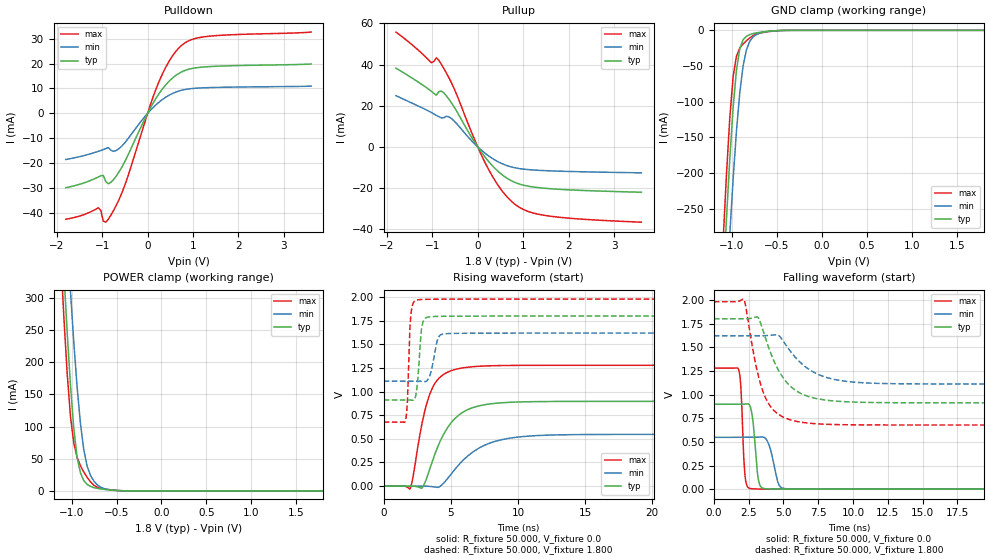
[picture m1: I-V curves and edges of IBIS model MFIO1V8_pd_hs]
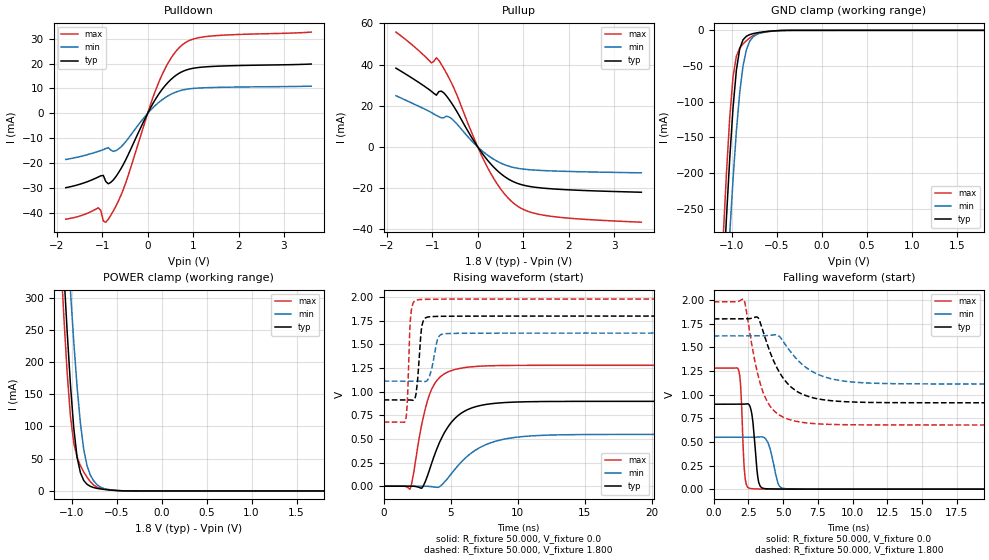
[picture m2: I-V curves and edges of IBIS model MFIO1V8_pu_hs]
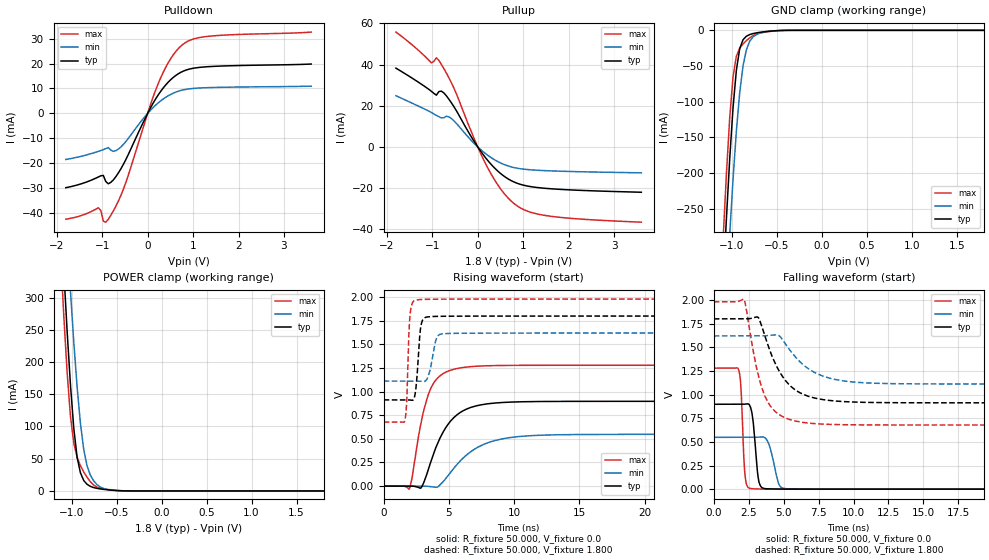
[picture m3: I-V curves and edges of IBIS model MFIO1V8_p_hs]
| IBIS file lpc55s6x_vfbga98.ibs
[IBIS Ver]   5.0
[File name]   lpc55s6x_vfbga98.ibs
[File Rev]   1.0
[Date]   May 25,2020
[Notes]   Rev History
|   1.0  initial release
[Disclaimer]   The model given below represents a 98-pin package.
[Copyright]   Copyright NXP 2020
|   Component lpc55s6x:vfbga98
[Component] lpc55s6x
[Manufacturer] NXP
[Package]
|   typ   min   max
R_pkg   0.1209   0.044925   0.28644
L_pkg   2.048e-9   9.518e-10   5.863e-9
C_pkg   3.001e-13   1.858e-13   5.678e-13
[Pin]   Signal_name   model_name   R_pin   L_pin   C_pin
G2   VDDA   POWER   NA   NA   NA
N7   USB1_3V3   POWER   NA   NA   NA
A3   USB0_3V3   POWER   NA   NA   NA
A5   VDD   POWER   NA   NA   NA
A9   VDD   POWER   NA   NA   NA
A13   VDD   POWER   NA   NA   NA
M1   VDD   POWER   NA   NA   NA
M9   VDD_PMU   POWER   NA   NA   NA
N6   USB1_DM   NC   0.094006   1.426e-9   2.165e-13
M6   USB1_DP   NC   0.094615   1.516e-9   2.317e-13
N9   FB   NC   0.12218   1.681e-9   2.209e-13
N11   LX   NC   0.06538   1.432e-9   3.1e-13
L12   P0_0   gpio1v8   0.094413   1.591e-9   2.392e-13
F5   P0_1   gpio1v8   0.09009   1.63e-9   3.407e-13
B11   P0_2   gpio1v8   0.10271   1.839e-9   2.924e-13
F8   P0_3   gpio1v8   0.1454   2.708e-9   3.901e-13
E7   P0_4   gpio1v8   0.091626   1.515e-9   3.275e-13
A7   P0_5   gpio1v8   0.12923   2.076e-9   2.188e-13
B7   P0_6   gpio1v8   0.11077   1.654e-9   2.153e-13
G5   P0_7   gpio1v8   0.13963   2.496e-9   4.691e-13
M2   P0_8   gpio1v8   0.095249   1.692e-9   2.933e-13
L13   P0_9   gpio1v8   0.15164   2.569e-9   2.247e-13
F2   P0_10   gpio1v8   0.12482   2.207e-9   3.527e-13
F1   P0_11   gpio1v8   0.13661   2.235e-9   2.226e-13
E2   P0_12   gpio1v8   0.10697   1.857e-9   3.137e-13
C12   P0_13   iicgpio1v8   0.15036   2.528e-9   2.486e-13
C13   P0_14   iicgpio1v8   0.15468   2.443e-9   2.364e-13
L2   P0_15   gpio1v8   0.098205   1.674e-9   2.761e-13
J2   P0_16   gpio1v8   0.12449   2.514e-9   2.708e-13
G3   P0_17   gpio1v8   0.075726   1.285e-9   2.687e-13
H9   P0_18   gpio1v8   0.087847   1.562e-9   3.542e-13
E6   P0_19   gpio1v8   0.083442   1.458e-9   2.858e-13
B12   P0_20   gpio1v8   0.14629   2.14e-9   2.464e-13
A12   P0_21   gpio1v8   0.12809   1.906e-9   1.918e-13
E9   P0_22   gpio1v8   0.094505   1.588e-9   3.718e-13
J1   P0_23   gpio1v8   0.13195   1.94e-9   2.141e-13
E12   P0_24   gpio1v8   0.091918   1.666e-9   2.453e-13
A11   P0_25   gpio1v8   0.11529   1.718e-9   1.949e-13
H12   P0_26   gpio1v8   0.081253   1.5e-9   2.767e-13
N2   P0_27   gpio1v8   0.13095   2.225e-9   3.428e-13
F13   P0_28   gpio1v8   0.13767   2.192e-9   2.158e-13
H8   P0_29   gpio1v8   0.15886   3.15e-9   5.678e-13
E5   P0_30   gpio1v8   0.086667   1.519e-9   3.383e-13
L1   P0_31   gpio1v8   0.15272   2.424e-9   2.59e-13
E1   P1_0   gpio1v8   0.14644   2.463e-9   2.597e-13
G11   P1_1   gpio1v8   0.096065   1.69e-9   3.188e-13
G12   P1_2   gpio1v8   0.12798   2.099e-9   2.352e-13
G13   P1_3   gpio1v8   0.12828   1.937e-9   2.153e-13
B2   P1_4   gpio1v8   0.096863   1.598e-9   2.988e-13
M5   P1_5   gpio1v8   0.094289   1.603e-9   3.053e-13
H5   P1_6   gpio1v8   0.16673   3.191e-9   4.881e-13
J5   P1_7   gpio1v8   0.12619   2.354e-9   3.979e-13
A6   P1_8   gpio1v8   0.28644   5.863e-9   4.62e-13
C1   P1_9   gpio1v8   0.1694   3.073e-9   3.031e-13
J7   P1_10   gpio1v8   0.08793   1.355e-9   3.087e-13
G6   P1_11   gpio1v8   0.15151   2.536e-9   5.272e-13
F12   P1_12   gpio1v8   0.082887   1.462e-9   2.268e-13
B3   P1_13   gpio1v8   0.11404   1.893e-9   2.97e-13
L7   P1_14   gpio1v8   0.18217   3.548e-9   3.635e-13
B6   P1_15   gpio1v8   0.12901   2.443e-9   3.381e-13
C7   P1_16   gpio1v8   0.072915   1.186e-9   2.322e-13
J9   P1_17   gpio1v8   0.10787   1.748e-9   3.803e-13
G9   P1_18   gpio1v8   0.091968   1.458e-9   3.094e-13
H13   P1_19   gpio1v8   0.12429   2.047e-9   2.027e-13
C2   P1_20   gpio1v8   0.096736   1.471e-9   2.029e-13
M7   P1_21   gpio1v8   0.14632   2.946e-9   3.43e-13
M8   P1_22   gpio1v8   0.076897   1.014e-9   2.527e-13
J8   P1_23   gpio1v8   0.085096   1.345e-9   3.077e-13
F6   P1_24   gpio1v8   0.13441   2.357e-9   4.172e-13
B8   P1_25   gpio1v8   0.10461   2.067e-9   3.287e-13
E13   P1_26   gpio1v8   0.12992   1.953e-9   2.102e-13
E8   P1_27   gpio1v8   0.11191   1.807e-9   3.572e-13
A8   P1_28   gpio1v8   0.21716   4.383e-9   3.836e-13
G8   P1_29   gpio1v8   0.15479   2.956e-9   4.522e-13
F9   P1_30   gpio1v8   0.093936   1.556e-9   3.54e-13
H6   P1_31   gpio1v8   0.14695   2.973e-9   5.442e-13
J6   RESETN   gpio1v8   0.08999   1.312e-9   3.328e-13
A1   USB0_DM   NC   0.17463   2.687e-9   2.917e-13
A2   USB0_DP   NC   0.16587   2.364e-9   2.831e-13
N13   VBAT_DCDC   NC   0.044925   1.39e-9   3.067e-13
M13   VBAT_PMU   NC   0.11627   1.679e-9   2.076e-13
N8   VBUS   NC   0.076519   9.518e-10   1.858e-13
H1   VREFN   NC   0.12485   1.889e-9   2.171e-13
G1   VREFP   NC   0.12475   1.856e-9   2.204e-13
J12   XTAL32K_N   NC   0.11411   1.691e-9   2.046e-13
J13   XTAL32K_P   NC   0.13248   1.96e-9   2.273e-13
M3   XTAL32M_N   NC   0.15178   2.164e-9   3.058e-13
N3   XTAL32M_P   NC   0.14758   1.994e-9   3.19e-13
B5   VSS   GND   NA   NA   NA
B9   VSS   GND   NA   NA   NA
B13   VSS   GND   NA   NA   NA
N1   VSS   GND   NA   NA   NA
H2   VSSA   GND   NA   NA   NA
N5   USB1_VSS   GND   NA   NA   NA
N12   VSS_DCDC   GND   NA   NA   NA
M12   VSS_DCDC   GND   NA   NA   NA
M11   VSS_PMU   GND   NA   NA   NA
B1   USB0_VSS   GND   NA   NA   NA
|   Model Selector
[Model Selector] gpio1v8
MFIO1V8_pd_hs  EPUN=1 EPD=1 EHS=1
MFIO1V8_pd_ls  EPUN=1 EPD=1 EHS=0
MFIO1V8_pu_hs  EPUN=0 EPD=0 EHS=1
MFIO1V8_pu_ls  EPUN=0 EPD=0 EHS=0
MFIO1V8_p_hs  EPUN=1 EPD=0 EHS=1
MFIO1V8_p_ls  EPUN=1 EPD=0 EHS=0
MFIO1V8_r_hs  EPUN=0 EPD=1 EHS=1
MFIO1V8_r_ls  EPUN=0 EPD=1 EHS=0
[Model Selector] iicgpio1v8
IIC1V8_pd_hs  EGP=1 EPUN=1 EPD=1 EHS=1
IIC1V8_pd_ls  EGP=1 EPUN=1 EPD=1 EHS=0
IIC1V8_p_hs  EGP=1 EPUN=1 EPD=0 EHS=1
IIC1V8_p_ls  EGP=1 EPUN=1 EPD=0 EHS=0
IIC1V8_pu_hs  EGP=1 EPUN=0 EPD=0 EHS=1
IIC1V8_pu_ls  EGP=1 EPUN=0 EPD=0 EHS=0
IIC1V8_r_hs  EGP=1 EPUN=0 EPD=1 EHS=1
IIC1V8_r_ls  EGP=1 EPUN=0 EPD=1 EHS=0
IIC1V8_pd_iic_hs  EGP=0 ECS=0 EPUN=1 EPD=1
IIC1V8_p_iic_hs  EGP=0 ECS=0 EPUN=1 EPD=0
IIC1V8_pu_iic_hs  EGP=0 ECS=0 EPUN=0 EPD=0
IIC1V8_r_iic_hs  EGP=0 ECS=0 EPUN=0 EPD=1
IIC1V8_pd_iic_pu_hs  EGP=0 ECS=1 EPUN=1 EPD=1  SSEL=1
IIC1V8_p_iic_pu_hs  EGP=0 ECS=1 EPUN=1 EPD=0  SSEL=1
IIC1V8_pu_iic_pu_hs  EGP=0 ECS=1 EPUN=0 EPD=0  SSEL=1
IIC1V8_r_iic_pu_hs  EGP=0 ECS=1 EPUN=0 EPD=1  SSEL=1
| Models and submodels in the file (24): MFIO1V8_pd_hs (I/O), MFIO1V8_pd_ls (I/O), MFIO1V8_pu_hs (I/O), MFIO1V8_pu_ls (I/O), MFIO1V8_p_hs (I/O), MFIO1V8_p_ls (I/O), MFIO1V8_r_hs (I/O), MFIO1V8_r_ls (I/O), IIC1V8_pd_hs (I/O), IIC1V8_pd_ls (I/O), IIC1V8_p_hs (I/O), IIC1V8_p_ls (I/O), IIC1V8_pu_hs (I/O), IIC1V8_pu_ls (I/O), IIC1V8_r_hs (I/O), IIC1V8_r_ls (I/O), IIC1V8_pd_iic_hs (I/O_open_drain), IIC1V8_p_iic_hs (I/O_open_drain), IIC1V8_pu_iic_hs (I/O_open_drain), IIC1V8_r_iic_hs (I/O_open_drain), IIC1V8_pd_iic_pu_hs (I/O_open_drain), IIC1V8_p_iic_pu_hs (I/O_open_drain), IIC1V8_pu_iic_pu_hs (I/O_open_drain), IIC1V8_r_iic_pu_hs (I/O_open_drain)
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|   Model MFIO1V8_pd_hs
[Model] MFIO1V8_pd_hs
Model_type I/O
Polarity   Non-Inverting
Enable   Active-Low
Vinl =  0.540V
Vinh =  1.260V
Vmeas =  0.900V
Cref =  0.0F
Rref =  100.000
Vref =  0.0V
C_comp   2.019pF   1.989pF   2.068pF
C_comp_pullup   1.198pF   1.161pF   1.251pF
C_comp_pulldown   0.670pF   0.661pF   0.684pF
[Model Spec]
Vinh   1.260V   1.134V   1.386V
Vinl   0.540V   0.486V   0.594V
Vmeas   0.900V   0.810V   0.990V
Vref   0.0V   0.0V   0.0V
Cref   0.0F   0.0F   0.0F
Rref   100.000   100.000   100.000
[Temperature Range]   25.000   0.125k   -40.000
[Voltage Range]   1.800V   1.620V   1.980V
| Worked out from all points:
|   slope of the pulldown table from 0 to 0.27 V, typ, clamps not added: 32.2 ohm
|   slope of the pullup table from 0 to 0.27 V, typ, clamps not added: 34.3 ohm
|   GND clamp passes 1 mA (typ) near -0.56 V on its own axis
|   POWER clamp passes 1 mA (typ) near -0.54 V on its own axis
|   rising waveform, R_fixture 50.000, V_fixture 0.0: 20-80 % time 1.89ns typ, 2.69ns min, 1.21ns max; typ from 0 V to 0.897 V
|   rising waveform, R_fixture 50.000, V_fixture 1.800: 20-80 % time 276ps typ, 422ps min, 194ps max; typ from 0.912 V to 1.8 V
|   falling waveform, R_fixture 50.000, V_fixture 0.0: 20-80 % time 315ps typ, 502ps min, 217ps max; typ from 0.897 V to 0 V
|   falling waveform, R_fixture 50.000, V_fixture 1.800: 20-80 % time 1.84ns typ, 2.3ns min, 1.28ns max; typ from 1.8 V to 0.912 V
[Pulldown]
|Voltage   I(typ)   I(min)   I(max)
-1.8V     -29.75mA   -18.45mA   -42.39mA
-1.085V   -25.48mA   -15.2mA    -37.79mA
-1.03V    -24.99mA   -14.87mA   -38.88mA
-975mV    -24.83mA   -14.51mA   -43.15mA
-865mV    -28.18mA   -13.68mA   -42.43mA
-700mV    -25.38mA   -14.92mA   -37.23mA
-480mV    -18.54mA   -11.29mA   -27.73mA
235mV     7.474mA    4.265mA    12.03mA
510mV     13.55mA    7.648mA    22.01mA
785mV     16.96mA    9.446mA    27.8mA
1.39V     18.81mA    10.38mA    31.01mA
3.6V      19.8mA     10.93mA    32.61mA
[Pullup]
|Voltage   I(typ)   I(min)   I(max)
-1.8V     38.29mA    24.9mA     55.82mA
-1.02V    27.05mA    16.71mA    40.87mA
-910mV    25.14mA    15.31mA    43.32mA
-855mV    26.89mA    14.69mA    42.04mA
-745mV    26.24mA    14.22mA    38.06mA
-580mV    21.45mA    13.82mA    31.22mA
190mV     -5.761mA   -3.564mA   -8.914mA
520mV     -13.24mA   -7.997mA   -20.92mA
795mV     -17.02mA   -10.03mA   -27.47mA
1.07V     -18.92mA   -10.95mA   -31.04mA
1.51V     -20.18mA   -11.56mA   -33.41mA
3.6V      -22.04mA   -12.6mA    -36.6mA
[GND_clamp]
|Voltage   I(typ)   I(min)   I(max)
-1.8V     -2.463A    -2.494A    -2.446A
-1.097V   -357.7mA   -460.7mA   -294.8mA
-1.06V    -264.9mA   -370.9mA   -202.5mA
-1.023V   -180.4mA   -286.3mA   -122.9mA
-986mV    -108.7mA   -208.9mA   -65.05mA
-949mV    -56.06mA   -141.4mA   -36.24mA
-912mV    -25.87mA   -87.65mA   -25.01mA
-875mV    -13.21mA   -49.99mA   -19.06mA
-838mV    -8.315mA   -27.44mA   -14.52mA
-764mV    -4.558mA   -9.219mA   -7.395mA
-542mV    -813.9uA   -810.7uA   -1.086mA
1.8V      0A         0A         0A
[POWER_clamp]
|Voltage   I(typ)   I(min)   I(max)
-1.8V     2.577A     2.626A     2.553A
-1.123V   442.8mA    582.7mA    371.8mA
-1.086V   342mA      487.8mA    272.2mA
-1.049V   248.2mA    396.7mA    184.1mA
-1.012V   164.7mA    310.5mA    115.9mA
-975mV    97.4mA     231.2mA    74.47mA
-938mV    52.21mA    161.5mA    52.2mA
-864mV    16.15mA    64.06mA    29.43mA
-790mV    7.073mA    24.26mA    14.23mA
-679mV    3.152mA    6.087mA    4.407mA
-494mV    590.1uA    655.5uA    758.5uA
1.8V      0A         0A         0A
[Ramp]
| variable   typ   min   max
dV/dt_r   0.538/1.890n   0.328/2.680n   0.767/1.209n
dV/dt_f   0.532/1.835n   0.305/2.291n   0.781/1.275n
R_load = 50.000
[Rising Waveform]
R_fixture= 50.000
V_fixture= 0.0
V_fixture_min= 0.0
V_fixture_max= 0.0
|time   V(typ)   V(min)   V(max)
0s        6.721nV    117.6nV    4.416nV
1.96ns    159.2uV    -62.09nV   -31.69mV
2.85ns    -21.07mV   134.7uV    661mV
3.65ns    271.3mV    -6.708mV   1.047V
4.15ns    457.1mV    -8.65mV    1.146V
4.97ns    661.3mV    117.8mV    1.218V
6.65ns    830.9mV    361.7mV    1.264V
9.15ns    884.8mV    501.2mV    1.276V
13.74ns   896.1mV    543.8mV    1.278V
100ns     896.7mV    547.4mV    1.278V
[Rising Waveform]
R_fixture= 50.000
V_fixture= 1.800
V_fixture_min= 1.620
V_fixture_max= 1.980
|time   V(typ)   V(min)   V(max)
0s        911.9mV    1.111V     677.7mV
1.63ns    911.9mV    1.111V     697.7mV
1.77ns    912.1mV    1.111V     900.3mV
2.05ns    909.6mV    1.111V     1.849V
2.42ns    983.6mV    1.111V     1.967V
2.68ns    1.419V     1.11V      1.973V
3.06ns    1.772V     1.105V     1.976V
4.08ns    1.796V     1.575V     1.978V
4.84ns    1.798V     1.614V     1.979V
100ns     1.799V     1.619V     1.979V
[Falling Waveform]
R_fixture= 50.000
V_fixture= 0.0
V_fixture_min= 0.0
V_fixture_max= 0.0
|time   V(typ)   V(min)   V(max)
0s        896.7mV    547.4mV    1.278V
1.79ns    896.7mV    547.4mV    1.258V
1.93ns    896.6mV    547.4mV    1.106V
2.24ns    898.4mV    547.4mV    142.2mV
2.74ns    796.7mV    547.3mV    4.509mV
3.2ns     100.7mV    550.1mV    1.658mV
3.81ns    3.552mV    517mV      778.9uV
4.65ns    1.171mV    54.78mV    345.8uV
5.34ns    645.9uV    3.088mV    186.5uV
100ns     14.3nV     131.2nV    8.877nV
[Falling Waveform]
R_fixture= 50.000
V_fixture= 1.800
V_fixture_min= 1.620
V_fixture_max= 1.980
|time   V(typ)   V(min)   V(max)
0s        1.799V     1.619V     1.979V
2.17ns    1.799V     1.619V     2.003V
3.18ns    1.813V     1.619V     1.21V
3.88ns    1.522V     1.623V     915.7mV
4.62ns    1.262V     1.626V     793.3mV
5.16ns    1.14V      1.527V     750mV
6.98ns    971mV      1.252V     694.9mV
9.25ns    925.2mV    1.144V     680.9mV
13.25ns   913mV      1.113V     677.9mV
100ns     911.9mV    1.111V     677.7mV
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|   Model MFIO1V8_pu_hs
[Model] MFIO1V8_pu_hs
Model_type I/O
Polarity   Non-Inverting
Enable   Active-Low
Vinl =  0.540V
Vinh =  1.260V
Vmeas =  0.900V
Cref =  0.0F
Rref =  100.000
Vref =  0.0V
C_comp   2.019pF   1.989pF   2.068pF
C_comp_pullup   1.197pF   1.159pF   1.249pF
C_comp_pulldown   0.671pF   0.662pF   0.686pF
[Model Spec]
Vinh   1.260V   1.134V   1.386V
Vinl   0.540V   0.486V   0.594V
Vmeas   0.900V   0.810V   0.990V
Vref   0.0V   0.0V   0.0V
Cref   0.0F   0.0F   0.0F
Rref   100.000   100.000   100.000
[Temperature Range]   25.000   0.125k   -40.000
[Voltage Range]   1.800V   1.620V   1.980V
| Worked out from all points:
|   slope of the pulldown table from 0 to 0.27 V, typ, clamps not added: 32.2 ohm
|   slope of the pullup table from 0 to 0.27 V, typ, clamps not added: 34.3 ohm
|   GND clamp passes 1 mA (typ) near -0.56 V on its own axis
|   POWER clamp passes 1 mA (typ) near -0.54 V on its own axis
|   rising waveform, R_fixture 50.000, V_fixture 0.0: 20-80 % time 1.89ns typ, 2.68ns min, 1.21ns max; typ from 0.001 V to 0.898 V
|   rising waveform, R_fixture 50.000, V_fixture 1.800: 20-80 % time 275ps typ, 425ps min, 197ps max; typ from 0.913 V to 1.8 V
|   falling waveform, R_fixture 50.000, V_fixture 0.0: 20-80 % time 314ps typ, 505ps min, 216ps max; typ from 0.898 V to 0.001 V
|   falling waveform, R_fixture 50.000, V_fixture 1.800: 20-80 % time 1.84ns typ, 2.3ns min, 1.27ns max; typ from 1.8 V to 0.913 V
[Pulldown]
|Voltage   I(typ)   I(min)   I(max)
-1.8V     -29.75mA   -18.45mA   -42.39mA
-1.085V   -25.48mA   -15.2mA    -37.79mA
-1.03V    -24.99mA   -14.87mA   -38.88mA
-975mV    -24.83mA   -14.51mA   -43.15mA
-865mV    -28.18mA   -13.68mA   -42.43mA
-700mV    -25.38mA   -14.92mA   -37.23mA
-480mV    -18.54mA   -11.29mA   -27.73mA
235mV     7.474mA    4.265mA    12.03mA
510mV     13.55mA    7.648mA    22.01mA
785mV     16.96mA    9.446mA    27.8mA
1.39V     18.81mA    10.38mA    31.01mA
3.6V      19.8mA     10.93mA    32.61mA
[Pullup]
|Voltage   I(typ)   I(min)   I(max)
-1.8V     38.29mA    24.9mA     55.82mA
-1.02V    27.05mA    16.71mA    40.87mA
-910mV    25.14mA    15.31mA    43.32mA
-855mV    26.89mA    14.69mA    42.04mA
-745mV    26.24mA    14.22mA    38.06mA
-580mV    21.45mA    13.82mA    31.22mA
190mV     -5.761mA   -3.564mA   -8.914mA
520mV     -13.24mA   -7.997mA   -20.92mA
795mV     -17.02mA   -10.03mA   -27.47mA
1.07V     -18.92mA   -10.95mA   -31.04mA
1.51V     -20.18mA   -11.56mA   -33.41mA
3.6V      -22.04mA   -12.6mA    -36.6mA
[GND_clamp]
|Voltage   I(typ)   I(min)   I(max)
-1.8V     -2.463A    -2.494A    -2.446A
-1.097V   -357.7mA   -460.7mA   -294.9mA
-1.06V    -264.9mA   -371mA     -202.6mA
-1.023V   -180.4mA   -286.4mA   -122.9mA
-986mV    -108.7mA   -208.9mA   -65.09mA
-949mV    -56.09mA   -141.5mA   -36.28mA
-912mV    -25.91mA   -87.68mA   -25.06mA
-875mV    -13.24mA   -50.02mA   -19.11mA
-838mV    -8.35mA    -27.47mA   -14.57mA
-764mV    -4.593mA   -9.247mA   -7.441mA
-542mV    -849.5uA   -838.5uA   -1.132mA
1.8V      0A         0A         0A
[POWER_clamp]
|Voltage   I(typ)   I(min)   I(max)
-1.8V     2.577A     2.626A     2.553A
-1.123V   442.8mA    582.7mA    371.7mA
-1.086V   342mA      487.8mA    272.2mA
-1.049V   248.2mA    396.7mA    184.1mA
-1.012V   164.7mA    310.5mA    115.9mA
-975mV    97.36mA    231.1mA    74.42mA
-938mV    52.18mA    161.5mA    52.15mA
-864mV    16.11mA    64.03mA    29.39mA
-790mV    7.037mA    24.23mA    14.18mA
-679mV    3.116mA    6.059mA    4.361mA
-494mV    554.4uA    627.7uA    712.3uA
1.8V      0A         0A         0A
[Ramp]
| variable   typ   min   max
dV/dt_r   0.538/1.890n   0.329/2.680n   0.767/1.209n
dV/dt_f   0.532/1.835n   0.305/2.290n   0.781/1.276n
R_load = 50.000
[Rising Waveform]
R_fixture= 50.000
V_fixture= 0.0
V_fixture_min= 0.0
V_fixture_max= 0.0
|time   V(typ)   V(min)   V(max)
0s        630.6uV    679.1uV    587.5uV
1.96ns    789.2uV    678.8uV    -30.05mV
2.85ns    -19.7mV    812.3uV    661.1mV
3.62ns    261mV      -5.421mV   1.04V
4.13ns    453.5mV    -9.012mV   1.145V
4.91ns    652mV      107.5mV    1.216V
6.6ns     829.9mV    358mV      1.264V
9.06ns    885.4mV    500.2mV    1.277V
13.76ns   897.4mV    545.1mV    1.28V
100ns     898mV      548.7mV    1.28V
[Rising Waveform]
R_fixture= 50.000
V_fixture= 1.800
V_fixture_min= 1.620
V_fixture_max= 1.980
|time   V(typ)   V(min)   V(max)
0s        913.3mV    1.112V     678.9mV
1.63ns    913.3mV    1.112V     698.4mV
1.75ns    913.5mV    1.112V     853.9mV
2.02ns    911.7mV    1.112V     1.814V
2.4ns     967.4mV    1.112V     1.968V
2.67ns    1.397V     1.111V     1.974V
3.06ns    1.773V     1.107V     1.977V
4.07ns    1.797V     1.574V     1.979V
4.83ns    1.798V     1.615V     1.98V
100ns     1.8V       1.62V      1.98V
[Falling Waveform]
R_fixture= 50.000
V_fixture= 0.0
V_fixture_min= 0.0
V_fixture_max= 0.0
|time   V(typ)   V(min)   V(max)
0s        898mV      548.7mV    1.28V
1.79ns    898mV      548.7mV    1.259V
1.93ns    897.9mV    548.6mV    1.108V
2.24ns    899.8mV    548.7mV    143.9mV
2.76ns    775.9mV    548.5mV    5.275mV
3.23ns    78.56mV    551.7mV    2.369mV
3.84ns    4.35mV     511.3mV    1.439mV
4.67ns    1.941mV    48.66mV    967uV
5.32ns    1.374mV    4.206mV    798.7uV
100ns     630.7uV    679.1uV    587.5uV
[Falling Waveform]
R_fixture= 50.000
V_fixture= 1.800
V_fixture_min= 1.620
V_fixture_max= 1.980
|time   V(typ)   V(min)   V(max)
0s        1.8V       1.62V      1.98V
2.16ns    1.8V       1.62V      2.006V
3.18ns    1.814V     1.62V      1.212V
3.84ns    1.538V     1.623V     928.3mV
4.62ns    1.264V     1.627V     794.8mV
5.16ns    1.142V     1.528V     751.1mV
7.03ns    970.5mV    1.249V     695.5mV
9.17ns    927.3mV    1.147V     682.3mV
13.26ns   914.4mV    1.115V     679mV
100ns     913.3mV    1.112V     678.9mV
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|   Model MFIO1V8_p_hs
[Model] MFIO1V8_p_hs
Model_type I/O
Polarity   Non-Inverting
Enable   Active-Low
Vinl =  0.540V
Vinh =  1.260V
Vmeas =  0.900V
Cref =  0.0F
Rref =  100.000
Vref =  0.0V
C_comp   2.019pF   1.989pF   2.068pF
C_comp_pullup   1.197pF   1.160pF   1.250pF
C_comp_pulldown   0.671pF   0.662pF   0.686pF
[Model Spec]
Vinh   1.260V   1.134V   1.386V
Vinl   0.540V   0.486V   0.594V
Vmeas   0.900V   0.810V   0.990V
Vref   0.0V   0.0V   0.0V
Cref   0.0F   0.0F   0.0F
Rref   100.000   100.000   100.000
[Temperature Range]   25.000   0.125k   -40.000
[Voltage Range]   1.800V   1.620V   1.980V
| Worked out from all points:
|   slope of the pulldown table from 0 to 0.27 V, typ, clamps not added: 32.2 ohm
|   slope of the pullup table from 0 to 0.27 V, typ, clamps not added: 34.3 ohm
|   GND clamp passes 1 mA (typ) near -0.56 V on its own axis
|   POWER clamp passes 1 mA (typ) near -0.54 V on its own axis
|   rising waveform, R_fixture 50.000, V_fixture 0.0: 20-80 % time 1.89ns typ, 2.68ns min, 1.21ns max; typ from 0 V to 0.897 V
|   rising waveform, R_fixture 50.000, V_fixture 1.800: 20-80 % time 278ps typ, 422ps min, 192ps max; typ from 0.913 V to 1.8 V
|   falling waveform, R_fixture 50.000, V_fixture 0.0: 20-80 % time 314ps typ, 511ps min, 215ps max; typ from 0.897 V to 0 V
|   falling waveform, R_fixture 50.000, V_fixture 1.800: 20-80 % time 1.84ns typ, 2.3ns min, 1.28ns max; typ from 1.8 V to 0.913 V
[Pulldown]
|Voltage   I(typ)   I(min)   I(max)
-1.8V     -29.75mA   -18.45mA   -42.39mA
-1.085V   -25.48mA   -15.2mA    -37.79mA
-1.03V    -24.99mA   -14.87mA   -38.88mA
-975mV    -24.83mA   -14.51mA   -43.15mA
-865mV    -28.18mA   -13.68mA   -42.43mA
-700mV    -25.38mA   -14.92mA   -37.23mA
-480mV    -18.54mA   -11.29mA   -27.73mA
235mV     7.474mA    4.265mA    12.03mA
510mV     13.55mA    7.648mA    22.01mA
785mV     16.96mA    9.446mA    27.8mA
1.39V     18.81mA    10.38mA    31.01mA
3.6V      19.8mA     10.93mA    32.61mA
[Pullup]
|Voltage   I(typ)   I(min)   I(max)
-1.8V     38.29mA    24.9mA     55.82mA
-1.02V    27.05mA    16.71mA    40.87mA
-910mV    25.14mA    15.31mA    43.32mA
-855mV    26.89mA    14.69mA    42.04mA
-745mV    26.24mA    14.22mA    38.06mA
-580mV    21.45mA    13.82mA    31.22mA
190mV     -5.761mA   -3.564mA   -8.914mA
520mV     -13.24mA   -7.997mA   -20.92mA
795mV     -17.02mA   -10.03mA   -27.47mA
1.07V     -18.92mA   -10.95mA   -31.04mA
1.51V     -20.18mA   -11.56mA   -33.41mA
3.6V      -22.04mA   -12.6mA    -36.6mA
[GND_clamp]
|Voltage   I(typ)   I(min)   I(max)
-1.8V     -2.463A    -2.494A    -2.446A
-1.097V   -357.7mA   -460.7mA   -294.8mA
-1.06V    -264.9mA   -370.9mA   -202.5mA
-1.023V   -180.4mA   -286.3mA   -122.9mA
-986mV    -108.6mA   -208.9mA   -65.04mA
-949mV    -56.05mA   -141.4mA   -36.22mA
-912mV    -25.86mA   -87.64mA   -25mA
-875mV    -13.2mA    -49.98mA   -19.05mA
-838mV    -8.305mA   -27.43mA   -14.51mA
-764mV    -4.549mA   -9.211mA   -7.385mA
-542mV    -805.6uA   -803.8uA   -1.077mA
1.8V      0A         0A         0A
[POWER_clamp]
|Voltage   I(typ)   I(min)   I(max)
-1.8V     2.577A     2.626A     2.553A
-1.123V   442.8mA    582.7mA    371.7mA
-1.086V   342mA      487.8mA    272.1mA
-1.049V   248.2mA    396.6mA    184.1mA
-1.012V   164.7mA    310.5mA    115.9mA
-975mV    97.36mA    231.1mA    74.41mA
-938mV    52.17mA    161.5mA    52.14mA
-864mV    16.1mA     64.02mA    29.38mA
-790mV    7.028mA    24.22mA    14.17mA
-679mV    3.108mA    6.053mA    4.351mA
-494mV    546.6uA    621.4uA    702.9uA
1.8V      0A         0A         0A
[Ramp]
| variable   typ   min   max
dV/dt_r   0.538/1.892n   0.329/2.683n   0.768/1.210n
dV/dt_f   0.532/1.838n   0.305/2.294n   0.781/1.277n
R_load = 50.000
[Rising Waveform]
R_fixture= 50.000
V_fixture= 0.0
V_fixture_min= 0.0
V_fixture_max= 0.0
|time   V(typ)   V(min)   V(max)
0s        7.051nV    120nV      4.667nV
1.96ns    159.3uV    -60nV      -31.77mV
2.85ns    -21.07mV   134.7uV    659.8mV
3.66ns    277.4mV    -6.745mV   1.05V
4.15ns    457.5mV    -8.707mV   1.146V
5.02ns    670.7mV    126mV      1.221V
6.67ns    832.3mV    364.4mV    1.265V
9.24ns    886mV      503.8mV    1.277V
13.74ns   896.7mV    544.2mV    1.279V
100ns     897.3mV    547.8mV    1.279V
[Rising Waveform]
R_fixture= 50.000
V_fixture= 1.800
V_fixture_min= 1.620
V_fixture_max= 1.980
|time   V(typ)   V(min)   V(max)
0s        912.6mV    1.112V     678.1mV
1.63ns    912.6mV    1.112V     697.9mV
1.77ns    912.8mV    1.112V     903.5mV
2.03ns    910.9mV    1.112V     1.828V
2.4ns     967.2mV    1.112V     1.967V
2.66ns    1.375V     1.111V     1.974V
3ns       1.761V     1.107V     1.977V
4.06ns    1.797V     1.57V      1.979V
4.83ns    1.798V     1.615V     1.979V
100ns     1.8V       1.62V      1.98V
[Falling Waveform]
R_fixture= 50.000
V_fixture= 0.0
V_fixture_min= 0.0
V_fixture_max= 0.0
|time   V(typ)   V(min)   V(max)
0s        897.3mV    547.8mV    1.279V
1.79ns    897.3mV    547.8mV    1.258V
1.96ns    897.2mV    547.8mV    1.035V
2.25ns    899.3mV    547.8mV    128.7mV
2.75ns    785.4mV    547.7mV    4.896mV
3.23ns    77.6mV     550.8mV    1.878mV
3.83ns    3.769mV    511.9mV    959.3uV
4.67ns    1.371mV    47.13mV    456uV
5.37ns    779.8uV    3.194mV    261.7uV
100ns     14.63nV    133.6nV    9.13nV
[Falling Waveform]
R_fixture= 50.000
V_fixture= 1.800
V_fixture_min= 1.620
V_fixture_max= 1.980
|time   V(typ)   V(min)   V(max)
0s        1.8V       1.62V      1.98V
2.16ns    1.8V       1.62V      2.006V
3.19ns    1.813V     1.62V      1.204V
3.83ns    1.543V     1.623V     931.6mV
4.63ns    1.261V     1.626V     793.3mV
5.2ns     1.135V     1.52V      748.4mV
7.09ns    968mV      1.244V     694.1mV
9.25ns    926.1mV    1.145V     681.3mV
13.38ns   913.7mV    1.114V     678.3mV
100ns     912.6mV    1.112V     678.1mV
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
